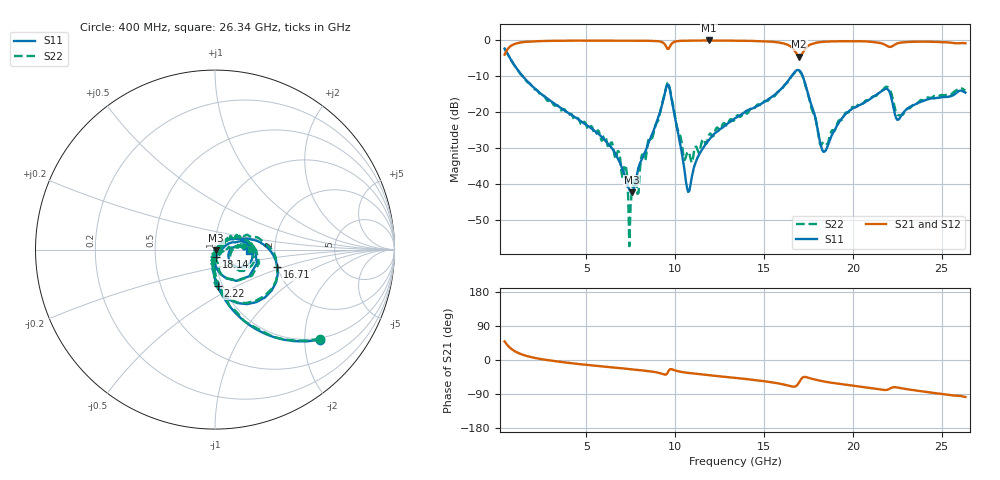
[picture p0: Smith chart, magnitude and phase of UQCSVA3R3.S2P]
!  Part Number  UQCSVA3R3  Mounting Orientation: Horizontal
!  Description: Ultra Low ESR Microwave capacitors
!  Application: Coupling, Bypass, Tuning, DC Block
!  Filters, Matching
# GHZ S DB R 50
! Freq  |S11|  S11 Ph  |S21|  S21 Ph  |S12|  S12 Ph  |S22|  S22 Ph
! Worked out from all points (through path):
!   400 points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, 400 MHz to 26.34 GHz, reference 50 ohm
!   highest |S21| = -0.01 dB at 11.9 GHz (marker M1); lowest = -4.5 dB at 16.98 GHz (marker M2)
!   group delay of S21, straight-line fit = 11.2 ps
!   lowest |S11| = -42.2 dB at 7.55 GHz (marker M3), VSWR 1.02, Z = 50.7 - j0.337 ohm
!   |S11| at or under -10 dB: 1.43 GHz to 16.54 GHz (15.11 GHz wide, 168 % of centre); 17.18 GHz to end of sweep
!   |S22| runs from -57.1 to -2.3 dB; largest |S21 - S12| = 0.0067
!   S11 on the Smith chart (normalised r, x): 400 MHz: 0.95, -2.37; 2.22 GHz: 0.95, -0.40; 16.71 GHz: 2.00, -0.45; 18.14 GHz: 1.01, -0.08; 26.34 GHz: 1.46, -0.03
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0.4  -2.25 -40.6  -3.97 49.1  -3.97 48.9  -2.27 -40.3
2.22  -13.88 -85.5  -0.20 4.4  -0.22 4.4  -13.81 -84.9
4.755  -22.66 -101.3  -0.06 -11.5  -0.06 -11.5  -23.37 -104.3
7.225  -38.57 -78.1  -0.05 -23.1  -0.05 -23.1  -35.01 -97.7
7.355  -40.65 -62.1  -0.06 -23.6  -0.06 -23.7  -43.52 -55.2
7.42  -41.37 -50.0  -0.06 -24.0  -0.05 -24.0  -57.14 -105.1
7.55  -42.19 -25.3  -0.06 -24.5  -0.06 -24.6  -42.47 -99.3
7.94  -35.22 30.5  -0.07 -26.4  -0.07 -26.5  -42.37 18.2
8.135  -32.89 32.7  -0.07 -27.4  -0.07 -27.5  -31.70 36.9
9.045  -21.40 38.0  -0.21 -33.5  -0.22 -33.6  -22.23 42.1
9.63  -12.35 -38.1  -2.36 -28.4  -2.35 -28.5  -11.97 -35.3
10.475  -34.35 -86.0  -0.09 -32.4  -0.09 -32.5  -32.33 -55.7
10.735  -42.10 -28.2  -0.07 -34.1  -0.07 -34.1  -30.87 -27.7
11.905  -27.60 45.0  -0.01 -40.1  -0.01 -40.2  -26.25 26.7
13.4  -21.52 39.7  -0.08 -47.4  -0.09 -47.5  -21.43 36.9
16.715  -8.85 -15.6  -2.80 -70.2  -2.80 -70.5  -9.03 -12.9
16.975  -8.28 -43.7  -4.48 -59.1  -4.50 -59.3  -8.44 -42.6
17.69  -18.32 -90.9  -1.00 -49.7  -1.00 -49.9  -19.07 -91.7
18.145  -28.04 -80.7  -0.47 -54.6  -0.47 -55.0  -28.65 -76.2
22.045  -14.10 -26.9  -1.79 -76.6  -1.81 -76.9  -13.49 -29.7
22.5  -22.05 -17.8  -0.84 -72.5  -0.87 -72.8  -20.68 -32.4
26.335  -14.48 -3.1  -0.79 -97.6  -0.81 -97.9  -13.90 1.5
